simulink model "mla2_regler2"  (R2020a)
settings: Solver=ode5  StartTime=0.0  StopTime=1  FixedStep=0.0001  RelTol=1e-4  EnableMultiTasking=on
PreLoadFcn:
  | MLA_Sensor1 = load('mla_sensor1.dat');
libraries: libmla x1, simulink_need_slupdate x1

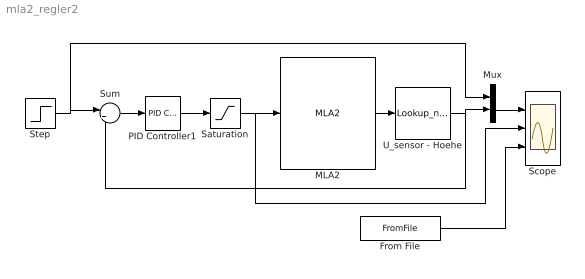
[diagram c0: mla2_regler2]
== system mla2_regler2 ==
  From File : FromFile  FileName=mla_regler2.mat  SampleTime=0
  MLA2 : libmla/MLA2  g=9.81  m=0.125  Fr_g=0.14  Fr_h=0.1  d_l=0.18  d_t=0.1  a=40691  b=0.0687  N=4.282
  Mux : Mux  Inputs=2
  PID Controller1 : simulink_need_slupdate/PID Controller  P=9000  I=2000  D=100
  Saturation : Saturate  UpperLimit=3  LowerLimit=-3
  Scope : Scope  NumInputPorts=3
  Step : Step  Time=0.1  After=0.02  SampleTime=0
  Sum : Sum  Inputs=|+-
  U_sensor - Hoehe : Lookup_n-D  NumberOfTableDimensions=1  BreakpointsForDimension1=MLA_Sensor1(:,1)  Table=MLA_Sensor1(:,2)  RndMeth=Simplest
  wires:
  MLA2/1 -> U_sensor - Hoehe/1
  Mux/1 -> Scope/1
  Sum/1 -> PID Controller1/1
  Step/1 -> Sum/1, Mux/1
  U_sensor - Hoehe/1 -> Mux/2, Sum/2
  PID Controller1/1 -> Saturation/1
  Saturation/1 -> MLA2/1, Scope/2
  From File/1 -> Scope/3
